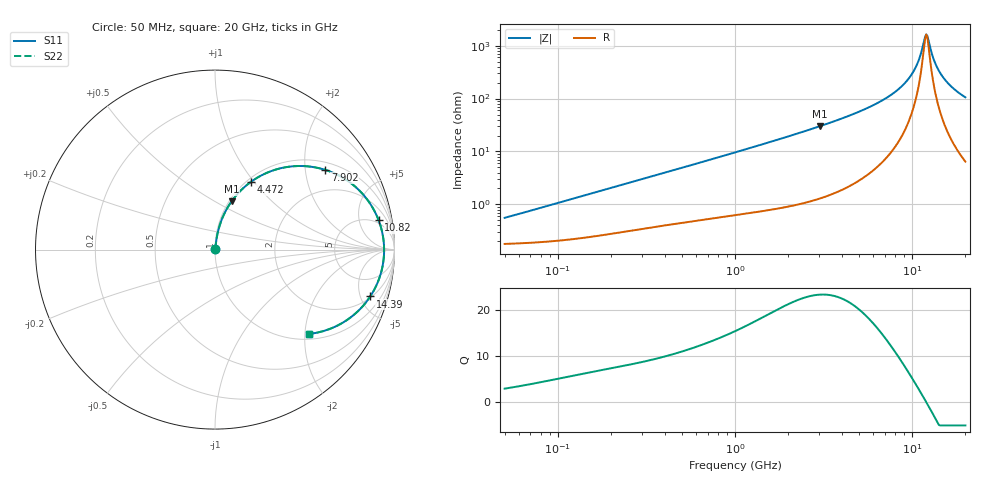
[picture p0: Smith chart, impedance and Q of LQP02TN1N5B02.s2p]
!Murata Part Number: LQP02TN1N5B02
!These Parameters are Measured in Series Mode Connection
!  o--[Z]--o
!Port1  Port2
!  o-------o
!Freq. Start=50[MHz] Stop=20[GHz], 401[Steps]
# Hz S RI R 50
!Freq.(Hz) S11(Real) S11(Imag) S21(Real) S21(Imag) S12(Real) S12(Imag) S22(Real) S22(Imag)
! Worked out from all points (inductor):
!   401 points, 50 MHz to 20 GHz, reference 50 ohm
!   read as one part in series: L = 1.68 nH near 51.52 MHz
!   highest Q = 23.2 at 3.03 GHz (marker M1), where L = 1.59 nH
!   self-resonance near 12.04 GHz
!   S11 on the Smith chart (normalised r, x): 50 MHz: 1.00, +0.01; 4.472 GHz: 1.05, +0.97; 7.902 GHz: 1.23, +2.57; 10.82 GHz: 4, +9; 14.39 GHz: 2.13, -6.05; 20 GHz: 1.13, -2.11
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5e7  0.00181 0.00526  0.9982 -0.00526  0.9982 -0.00526  0.00181 0.00526
1.364002e8  0.0025 0.0141  0.9975 -0.0141  0.9975 -0.0141  0.0025 0.0141
3.721004e8  0.00518 0.0365  0.9948 -0.0365  0.9948 -0.0365  0.00518 0.0365
1e9  0.0151 0.0938  0.9849 -0.0938  0.9849 -0.0938  0.0151 0.0938
2.728004e9  0.0766 0.2451  0.9234 -0.2451  0.9234 -0.2451  0.0766 0.2451
3.029571e9  0.0933 0.2701  0.9067 -0.2701  0.9067 -0.2701  0.0933 0.2701
4.472136e9  0.2003 0.3776  0.7997 -0.3776  0.7997 -0.3776  0.2003 0.3776
5.856089e9  0.3458 0.448  0.6542 -0.448  0.6542 -0.448  0.3458 0.448
7.442007e9  0.5517 0.4593  0.4483 -0.4593  0.4483 -0.4593  0.5517 0.4593
7.901521e9  0.614 0.4444  0.386 -0.4444  0.386 -0.4444  0.614 0.4444
8.774992e9  0.7274 0.3912  0.2726 -0.3912  0.2726 -0.3912  0.7274 0.3912
9.600142e9  0.8194 0.3135  0.1806 -0.3135  0.1806 -0.3135  0.8194 0.3135
1.019291e10  0.8717 0.2445  0.1283 -0.2445  0.1283 -0.2445  0.8717 0.2445
1.082228e10  0.9118 0.1634  0.0882 -0.1634  0.0882 -0.1634  0.9118 0.1634
1.115139e10  0.9261 0.1192  0.0739 -0.1192  0.0739 -0.1192  0.9261 0.1192
1.166392e10  0.9393 0.0499  0.0607 -0.0499  0.0607 -0.0499  0.9393 0.0499
1.201863e10  0.9422 0.0026  0.0578 -0.0026  0.0578 -0.0026  0.9422 0.0026
1.238412e10  0.9404 -0.0448  0.0596 0.0448  0.0596 0.0448  0.9404 -0.0448
1.334722e10  0.9155 -0.1593  0.0845 0.1593  0.0845 0.1593  0.9155 -0.1593
1.438523e10  0.8651 -0.2609  0.1349 0.2609  0.1349 0.2609  0.8651 -0.2609
1.646126e10  0.7337 -0.3934  0.2663 0.3934  0.2663 0.3934  0.7337 -0.3934
2e10  0.5255 -0.4698  0.4745 0.4698  0.4745 0.4698  0.5255 -0.4698
